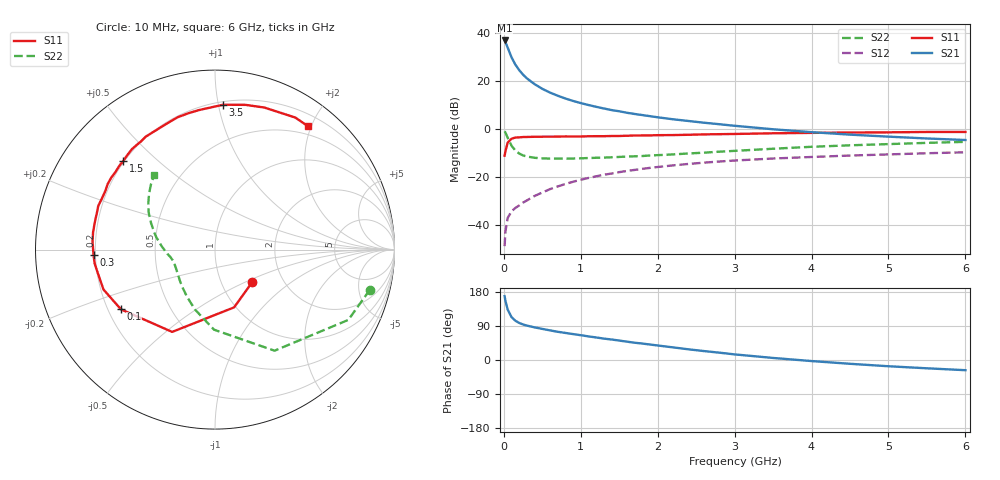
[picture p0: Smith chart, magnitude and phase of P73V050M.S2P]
! SIEMENS Small Signal Semiconductors
! BFP196
! Si NPN RF Bipolar Junction Transistor in SOT143
! VCE = 3 V  IC = 50 mA
! Common Emitter S-Parameters:  May  1996
# GHz  S  MA  R  50
!  f  S11  S21  S12  S22
! GHz  MAG  ANG  MAG  ANG  MAG  ANG  MAG  ANG
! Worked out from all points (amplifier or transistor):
!   36 points, 10 MHz to 6 GHz, reference 50 ohm
!   highest |S21| = 36.8 dB at 10 MHz (marker M1)
!   |S21| within 3 dB of that: start of sweep to 50.35 MHz
!   unconditionally stable (mu >= 1): 443.5 MHz to 4.195 GHz
!   at 250 MHz: K = 0.84, MSG = 26.6 dB, |S12| = -30.7 dB
!   at 1.4 GHz: K = 1.10, MAG = 11.3 dB, |S12| = -18.6 dB
!   at 6 GHz: K = 0.98, MSG = 2.6 dB, |S12| = -9.8 dB
!   S11 on the Smith chart (normalised r, x): 10 MHz: 1.39, -0.55; 100 MHz: 0.25, -0.27; 300 MHz: 0.19, -0.02; 1.5 GHz: 0.20, +0.39; 3.5 GHz: 0.22, +1.03; 6 GHz: 0.37, +1.95
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0.01  0.2757 -41.4  69.34 168.4  0.0036 80.3  0.8912 -14.6
0.02  0.339 -71.7  64.72 156.7  0.0072 70.7  0.8398 -27.8
0.05  0.517 -117.5  49.25 133.0  0.0139 55.5  0.6536 -59.5
0.1  0.6208 -147.6  30.89 113.2  0.0192 48.3  0.4462 -90.7
0.15  0.6599 -160.3  21.74 103.6  0.0225 48.9  0.3519 -108.5
0.2  0.6651 -168.1  16.69 97.8  0.0254 52.6  0.3058 -120.6
0.25  0.675 -173.4  13.41 93.7  0.0291 54.1  0.2791 -130.1
0.3  0.6773 -177.3  11.24 90.8  0.0323 56.6  0.2656 -136.3
0.4  0.6838 176.2  8.519 86.1  0.04 60.0  0.2494 -145.8
0.5  0.6862 171.8  6.819 82.1  0.0472 61.8  0.2425 -152.1
0.6  0.6867 166.9  5.694 78.2  0.0555 62.5  0.2403 -156.3
0.7  0.6889 162.9  4.896 74.5  0.0631 62.7  0.2396 -159.6
0.8  0.6946 159.5  4.284 71.4  0.0711 62.2  0.2403 -162.1
0.9  0.6914 155.6  3.812 68.4  0.0791 61.5  0.2408 -164.4
1.1  0.7006 148.6  3.136 62.3  0.0949 60.0  0.2466 -167.7
1.5  0.7106 136.1  2.322 51.3  0.1254 55.3  0.2599 -173.0
2.2  0.7418 116.2  1.582 33.3  0.1735 45.3  0.2936 177.4
2.8  0.7743 100.9  1.249 19.4  0.2084 36.6  0.3345 168.0
3.5  0.8083 86.8  0.98 5.4  0.2409 26.6  0.3851 157.6
4.5  0.8378 70.9  0.757 -10.0  0.2779 14.7  0.454 144.9
5.5  0.861 58.7  0.63 -21.9  0.3103 4.0  0.5103 134.3
6  0.8608 53.1  0.585 -26.9  0.325 -1.8  0.5359 129.1
